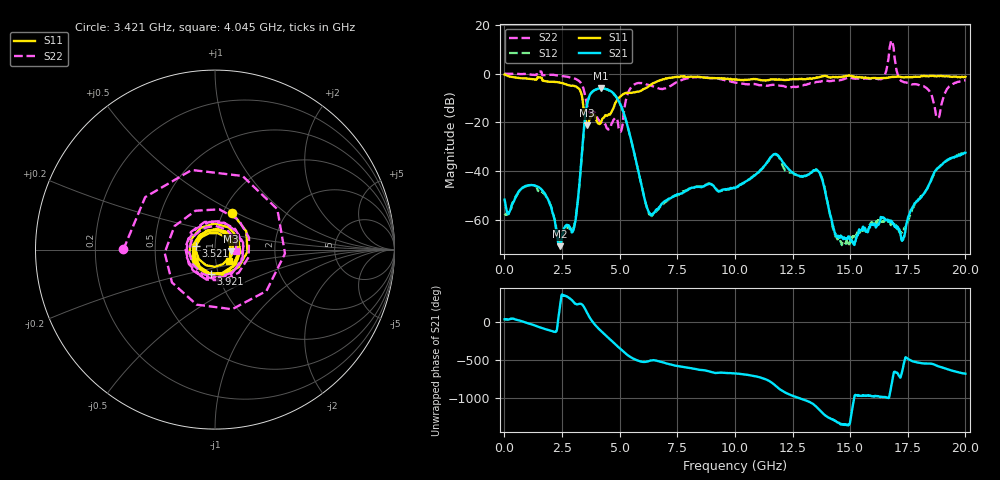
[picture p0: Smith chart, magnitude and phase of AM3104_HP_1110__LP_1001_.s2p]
!Created with skrf (http://scikit-rf.org).
# Hz S RI R 50.0
!freq ReS11 ImS11 ReS21 ImS21 ReS12 ImS12 ReS22 ImS22
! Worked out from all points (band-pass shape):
!   1601 points, 10 MHz to 20 GHz, reference 50 ohm
!   highest |S21| = -6.01 dB at 4.183 GHz (marker M1); lowest = -70.6 dB at 2.396 GHz (marker M2)
!   |S21| within 3 dB of the highest: 3.695 GHz to 4.818 GHz (1.122 GHz wide, 26.4 % of centre)
!   lowest |S11| = -21.1 dB at 3.596 GHz (marker M3), VSWR 1.19, Z = 59.6 - j1.04 ohm
!   |S11| at or under -10 dB: 3.38 GHz to 4.961 GHz (1.582 GHz wide, 37.9 % of centre)
!   |S22| runs from -23.8 to 13.5 dB; largest |S21 - S12| = 0.043
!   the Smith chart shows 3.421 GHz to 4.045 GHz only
!   S11 on the Smith chart (normalised r, x): 3.421 GHz: 1.10, +0.48; 3.521 GHz: 0.80, +0.04; 3.921 GHz: 0.92, -0.26; 4.045 GHz: 1.16, -0.14
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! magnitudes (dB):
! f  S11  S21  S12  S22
! 10 MHz  -0.4  -51.6  -58.0  0.0
! 1.297 GHz  -2.4  -45.7  -45.8  -0.6
! 2.396 GHz  -3.7  -70.6  -68.4  -0.9
! 3.021 GHz  -5.1  -63.0  -62.8  -1.9
! 3.346 GHz  -8.5  -34.8  -34.9  -4.2
! 3.421 GHz  -12.9  -25.7  -25.8  -5.8
! 3.521 GHz  -19.2  -16.4  -16.5  -9.8
! 3.596 GHz  -21.1  -12.1  -12.1  -13.5
! 3.921 GHz  -17.1  -6.8  -6.8  -15.9
! 4.045 GHz  -20.1  -6.2  -6.3  -18.4
! 4.183 GHz  -20.1  -6.0  -6.1  -19.9
! 5.008 GHz  -9.6  -12.1  -12.1  -23.4
! 6.219 GHz  -5.5  -55.7  -55.8  -4.6
! 6.682 GHz  -3.0  -55.2  -55.5  -6.0
! 10.01 GHz  -2.5  -46.9  -46.5  -3.7
! 11.72 GHz  -2.4  -33.0  -33.1  -4.6
! 13.34 GHz  -2.1  -40.3  -40.3  -3.9
! 14.58 GHz  -1.4  -67.0  -68.5  -2.7
! 16.68 GHz  -1.6  -60.4  -60.4  7.1
! 17.29 GHz  -1.5  -68.0  -64.5  -3.3
! 18.8 GHz  -1.0  -38.6  -38.8  -18.0
! 20 GHz  -1.4  -32.4  -31.8  -2.7
